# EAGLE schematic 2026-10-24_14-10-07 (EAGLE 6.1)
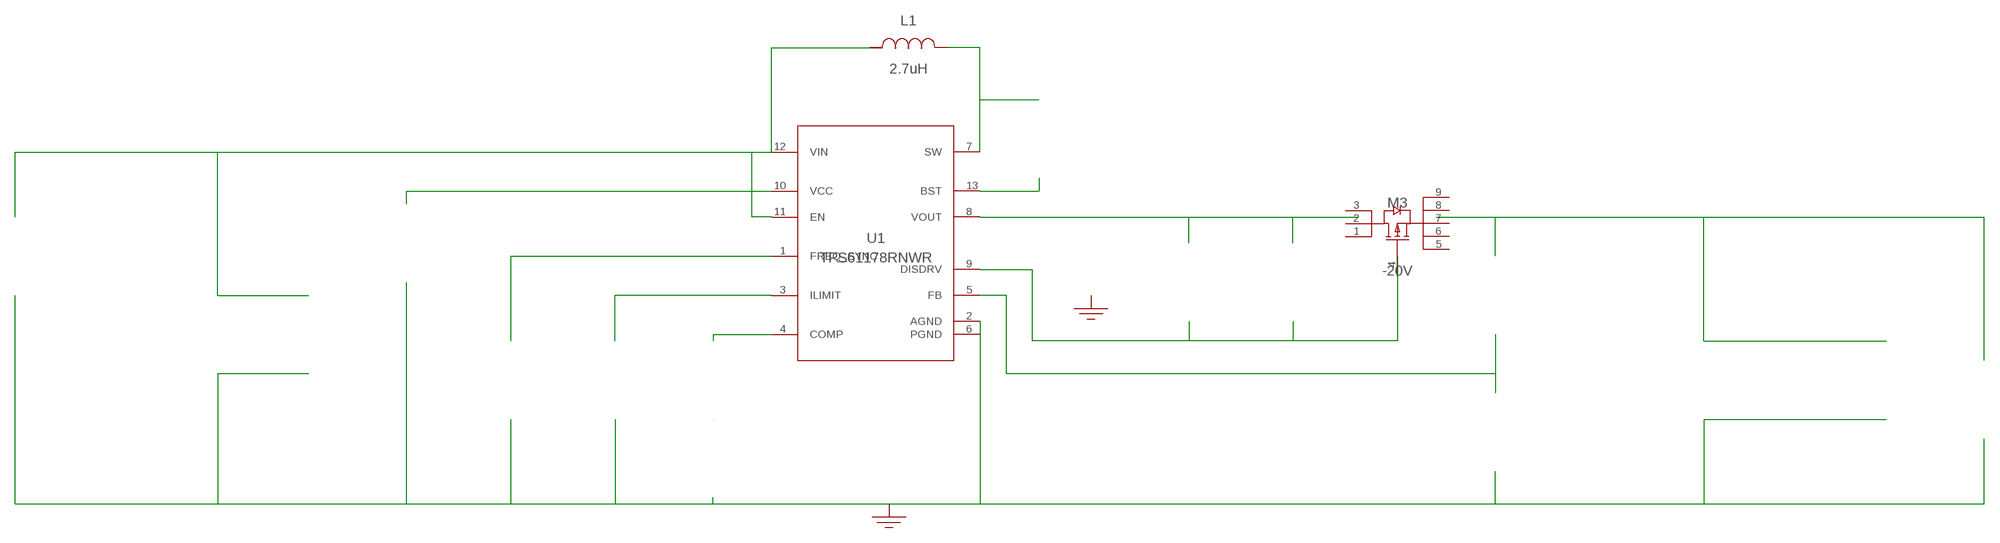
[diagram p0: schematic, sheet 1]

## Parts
CBOOT  100nF  08053C104KAT2A08053C104KAT2A  [0805]  (not placed on a sheet)
CCOMP  1.8nF  CL21C182JBF1PNECL21C182JBF1PNE  [0805]  (not placed on a sheet)
CGATE  22nF  C0805C223K5RACTUC0805C223K5RACTU  [0805]  (not placed on a sheet)
CIN  22uF  MSASE32MSB7226MPNB25MSASE32MSB7226MPNB25  [1210]  (not placed on a sheet)
CIN_2  22uF  MSASE32MSB7226MPNB25MSASE32MSB7226MPNB25  [1210]  (not placed on a sheet)
COUT  22uF  GRM32ER61E226KE15LGRM32ER61E226KE15L  [1210]  (not placed on a sheet)
COUT1  4.7uF  C3216X7R1E475K160ACC3216X7R1E475K160AC  [1206]  (not placed on a sheet)
COUT_2  22uF  GRM32ER61E226KE15LGRM32ER61E226KE15L  [1210]  (not placed on a sheet)
COUT_3  22uF  GRM32ER61E226KE15LGRM32ER61E226KE15L  [1210]  (not placed on a sheet)
CVCC  4.7uF  MSAST21GAB5475MTNA01MSAST21GAB5475MTNA01  [0805]  (not placed on a sheet)
GND  WB_GND  WB_GNDWB_GND  [WB_GND]
GND1  WB_GND  WB_GNDWB_GND  [WB_GND]
IOUT  WB_CURRENT_LOAD  WB_CURRENT_LOADWB_CURRENT_LOAD  [WB_CURRENT_LOAD]  (not placed on a sheet)
L1  2.7uH  1255AY-2R7N=P31255AY-2R7N=P3  [DG6045C]
M3  -20V  CSD25404Q3CSD25404Q3  [DQG0008A]
RCOMP  44.2k  CRCW020144K2FNEDCRCW020144K2FNED  [0201]  (not placed on a sheet)
RFBB  80.6k  CRCW040280K6FKEDCRCW040280K6FKED  [0402]  (not placed on a sheet)
RFBT  732k  CRCW0402732KFKEDCRCW0402732KFKED  [0402]  (not placed on a sheet)
RGATE  178k  CRCW0402178KFKEDCRCW0402178KFKED  [0402]  (not placed on a sheet)
RILIM  162k  RC0201FR-07162KLRC0201FR-07162KL  [0201]  (not placed on a sheet)
RT  169k  CRCW0402169KFKEDCRCW0402169KFKED  [0402]  (not placed on a sheet)
U1  TPS61178RNWR  TPS61178RNWRTPS61178RNWR  [RNW0013A]
VIN  WB_BATTERY  WB_BATTERYWB_BATTERY  [WB_BATTERY]  (not placed on a sheet)
Unconnected: CBOOT.1 CBOOT.2 CCOMP.1 CCOMP.2 CGATE.1 CGATE.2 CIN.1 CIN.2 CIN_2.1 CIN_2.2 COUT1.1 COUT1.2 COUT.1 COUT.2 COUT_2.1 COUT_2.2 COUT_3.1 COUT_3.2 CVCC.1 CVCC.2 GND1.1 GND.1 IOUT.1(+) IOUT.2(-) L1.1 L1.2 M3.1(D) M3.2(D) M3.3(D) M3.4(G) M3.5(S) M3.6(S) M3.7(S) M3.8(S) M3.9(S) RCOMP.1 RCOMP.2 RFBB.1 RFBB.2 RFBT.1 RFBT.2 RGATE.1 RGATE.2 RILIM.1 RILIM.2 RT.1 RT.2 U1.1(FREQ_SYNC) U1.3(ILIMIT) U1.4(COMP) U1.5(FB) U1.9(DISDRV) U1.11(EN) VIN.1(+) VIN.2(-)

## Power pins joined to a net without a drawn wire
AGND: U1.2(AGND)
BST: U1.13(BST)
PGND: U1.6(PGND)
SW: U1.7(SW)
VCC: U1.10(VCC)
VIN: U1.12(VIN)
VOUT: U1.8(VOUT)

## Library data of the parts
CBOOT = AcceleratedDesigns_Lib:08053C104KAT2A; Manufacturer_Part_Number: 08053C104KAT2A; Vendor: AVX
CCOMP = AcceleratedDesigns_Lib:CL21C182JBF1PNE; Manufacturer_Part_Number: CL21C182JBF1PNE; Vendor: Samsung Electro-Mechanics
CGATE = AcceleratedDesigns_Lib:C0805C223K5RACTU; Manufacturer_Part_Number: C0805C223K5RACTU; Vendor: Kemet
CIN CIN_2 = AcceleratedDesigns_Lib:MSASE32MSB7226MPNB25; Manufacturer_Part_Number: MSASE32MSB7226MPNB25; Vendor: Taiyo Yuden
COUT COUT_2 COUT_3 = AcceleratedDesigns_Lib:GRM32ER61E226KE15L; Manufacturer_Part_Number: GRM32ER61E226KE15L; Vendor: MuRata
COUT1 = AcceleratedDesigns_Lib:C3216X7R1E475K160AC; Manufacturer_Part_Number: C3216X7R1E475K160AC; Vendor: TDK
CVCC = AcceleratedDesigns_Lib:MSAST21GAB5475MTNA01; Manufacturer_Part_Number: MSAST21GAB5475MTNA01; Vendor: Taiyo Yuden
GND GND1 = AcceleratedDesigns_Lib:WB_GND; Manufacturer_Part_Number: WB_GND
IOUT = AcceleratedDesigns_Lib:WB_CURRENT_LOAD; Manufacturer_Part_Number: WB_CURRENT_LOAD
L1 = AcceleratedDesigns_Lib:1255AY-2R7N=P3; Manufacturer_Part_Number: 1255AY-2R7N=P3; Vendor: MuRata
M3 = AcceleratedDesigns_Lib:CSD25404Q3; Manufacturer_Part_Number: CSD25404Q3
RCOMP = AcceleratedDesigns_Lib:CRCW020144K2FNED; Manufacturer_Part_Number: CRCW020144K2FNED; Vendor: Vishay-Dale
RFBB = AcceleratedDesigns_Lib:CRCW040280K6FKED; Manufacturer_Part_Number: CRCW040280K6FKED; Vendor: Vishay-Dale
RFBT = AcceleratedDesigns_Lib:CRCW0402732KFKED; Manufacturer_Part_Number: CRCW0402732KFKED; Vendor: Vishay-Dale
RGATE = AcceleratedDesigns_Lib:CRCW0402178KFKED; Manufacturer_Part_Number: CRCW0402178KFKED; Vendor: Vishay-Dale
RILIM = AcceleratedDesigns_Lib:RC0201FR-07162KL; Manufacturer_Part_Number: RC0201FR-07162KL; Vendor: Yageo America
RT = AcceleratedDesigns_Lib:CRCW0402169KFKED; Manufacturer_Part_Number: CRCW0402169KFKED; Vendor: Vishay-Dale
U1 = AcceleratedDesigns_Lib:TPS61178RNWR; Manufacturer_Part_Number: TPS61178RNWR
VIN = AcceleratedDesigns_Lib:WB_BATTERY; Manufacturer_Part_Number: WB_BATTERY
